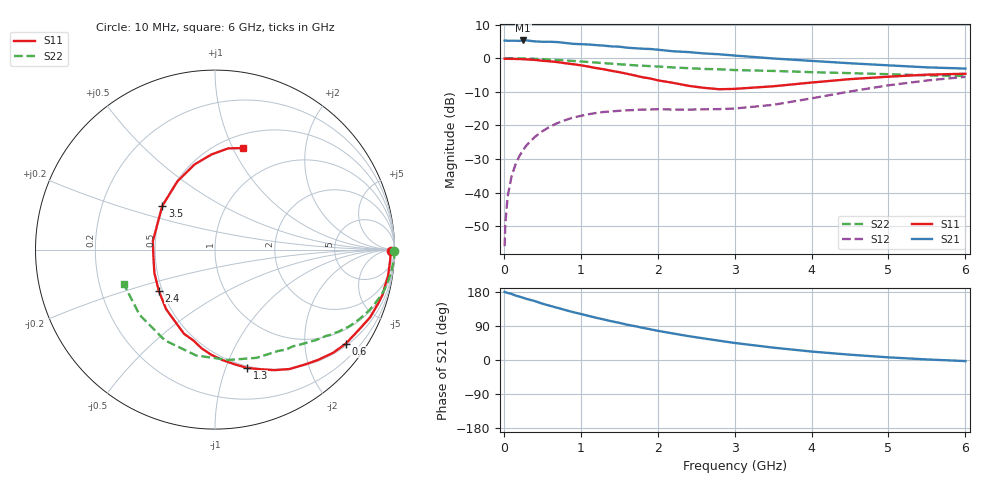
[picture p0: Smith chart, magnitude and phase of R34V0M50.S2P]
! SIEMENS Small Signal Semiconductors
! BFR181
! Si NPN RF Bipolar Junction Transistor in SOT23
! VCE = 4 V  IC = 0.5 mA
! Common Emitter S-Parameters:  May  1996
# GHz  S  MA  R  50
!  f  S11  S21  S12  S22
! GHz  MAG  ANG  MAG  ANG  MAG  ANG  MAG  ANG
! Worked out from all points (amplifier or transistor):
!   36 points, 10 MHz to 6 GHz, reference 50 ohm
!   highest |S21| = 5.3 dB at 250 MHz (marker M1)
!   |S21| within 3 dB of that: start of sweep to 2.107 GHz
!   unconditionally stable (mu >= 1): 2.378 GHz to 3.951 GHz
!   at 250 MHz: K = 0.12, MSG = 16.3 dB, |S12| = -27.3 dB
!   at 1.4 GHz: K = 0.61, MSG = 9.7 dB, |S12| = -15.8 dB
!   at 6 GHz: K = 0.92, MSG = 1.2 dB, |S12| = -5.5 dB
!   S11 on the Smith chart (normalised r, x): 10 MHz: 82, -47; 600 MHz: 0.56, -3.00; 1.3 GHz: 0.48, -1.19; 2.4 GHz: 0.48, -0.26; 3.5 GHz: 0.49, +0.28; 6 GHz: 0.63, +1.09
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0.01  0.9819 -0.6  1.822 179.7  0.0016 91.6  0.9999 -0.3
0.02  0.9778 -1.1  1.829 178.7  0.0036 87.0  0.9942 -0.6
0.05  0.9782 -3.0  1.814 177.1  0.0088 90.5  0.9987 -1.4
0.1  0.976 -5.9  1.817 174.3  0.0174 86.4  0.9997 -2.8
0.15  0.9751 -8.7  1.817 170.3  0.026 83.5  0.9955 -4.4
0.25  0.967 -15.0  1.834 164.3  0.0432 79.3  0.9915 -7.1
0.3  0.9584 -18.0  1.833 160.9  0.0514 77.8  0.9858 -8.5
0.4  0.943 -23.6  1.777 155.7  0.067 73.4  0.9782 -11.2
0.6  0.8973 -35.8  1.755 143.0  0.0959 65.7  0.9527 -16.5
0.8  0.8408 -47.0  1.684 131.8  0.12 58.3  0.9239 -21.4
1.1  0.7491 -63.7  1.599 116.5  0.1466 49.5  0.8769 -27.7
1.3  0.6828 -74.9  1.536 106.9  0.1585 44.5  0.8433 -31.5
1.5  0.6186 -85.8  1.482 98.1  0.1649 40.5  0.8114 -35.0
1.8  0.5207 -103.3  1.383 85.2  0.1723 36.6  0.7729 -39.3
2.2  0.4296 -129.3  1.266 70.0  0.172 34.1  0.7285 -45.4
2.4  0.388 -143.9  1.232 63.0  0.1718 34.6  0.7101 -48.2
3  0.3495 172.2  1.094 45.0  0.1783 40.7  0.6656 -58.0
3.5  0.3818 140.3  0.99 32.7  0.2021 47.3  0.646 -69.0
4.5  0.4878 103.6  0.84 14.0  0.3197 50.3  0.5992 -100.1
5  0.5305 92.1  0.782 7.0  0.3947 45.3  0.5775 -118.9
5.5  0.5687 82.6  0.73 1.5  0.4658 37.6  0.5555 -139.1
6  0.5865 74.7  0.7 -2.9  0.5284 28.9  0.5434 -159.4
